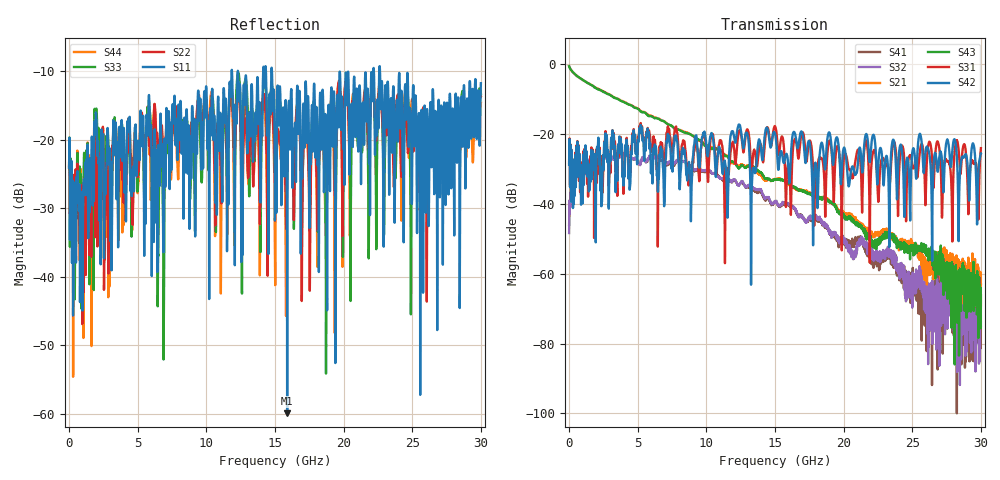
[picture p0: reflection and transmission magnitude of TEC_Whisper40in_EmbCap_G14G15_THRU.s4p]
! Tyco Electronics
! G14G15_THRU
!! PART DESCRIPTION: Whisper 40in Megtron 6 VLP-HVLP-VLP Channel, Embedded Capactior Connecter at one end, bulkhead 2.4mm test pts
!! MODEL DESCRIPTION: System 4-port S-parameter
!! MODEL STATUS: Measured
!! MODEL GEOMETRY: Channel Model
!! MODEL FREQUENCY RANGE: DC to 30.000 GHz in 10.000 MHz frequency steps
!! MODEL EDGE RATE LIMITATION: 12.500 ps (Using conservative 0.5/Fmax rule of thumb)
!! TIME-DOMAIN TRANSFORM CAUTIONS:
!! 1.) Do not simulate transient edge rates faster than the number listed above.  Edge rates faster than this number
!!  contain significant spectral content at frequencies above the model's highest frequency.
!! 2.) Even when simulating edge rates that are slower than the number listed above, be aware that the best time
!!  resolution possible with a direct iFFT is (1 / 2Fmax).  As a result, time resolution is typically not adequate
!!  for most time-domain simulations unless tricks such as windowing are used to minimize leakage and aliasing.
!! 3.) Because the model has a uniform frequency step, a direct iFFT will result in an impulse that that has a time
!!  length given by either (1 / Fstep) or (1 / 2Fstep), depending on the transform being used.  Care has been taken
!!  in selecting the frequency step to ensure a settled impulse response for the model.  Therefore, convolution with
!!  the model's impulse response should present no issues.  However, if directly concatenating s-parameter models
!!  in the frequency domain a user must either interpolate necessary interim frequencies or complete impulse response
!!  zero-padding.  Impulse response zero-padding is more difficult, but more accurate.
!! PORT DEFINITIONS:
!! Port  1  ----->  Side A  G14  Side B  <-----  Port  2
!! Port  3  ----->  Side A  G15  Side B  <-----  Port  4
! Point-to-Point link (differential)  !
! Connectors:  !
!  1: STRADA Whisper  !
! Materials:  !
!  Backplane: Megtron-6 HVLP  !
!  Daughtercard: Megtron-6 VLP  !
! Stack-up:  !
!  Backplane: 20 layers, 200mil thick  !
!  Daughtercard: 14 layers, 110mil thick  !
! Trace Length:  !
!  Backplane: 30in  !
!  Daightercards: 5in  !
! Trace Width:  !
!  Backplane: 7-9-7 mils  !
!  Daughtercards: 6-9-6 mils  !
! Geometry:  !
!  Backplane: Stripline  !
!  Daughtercards: Stripline  !
! Layer Connections:  !
!  Backplane: Layer 16, counterbored(~6mil stub)  !
!  Daughtercard: Layer 9, counterbored(~6mil stub)  !
! Freq. Range: 0 GHz - 30 GHz  !
! Note1: non-mixed-mode s-parameters  !
! Note2: channel includes 2.4mm test points  !
! Touchstone data
! Created: 02-Jul-2013 by IdEM R2011 (7.0.3)
# Hz S MA R 50
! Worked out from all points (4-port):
!   3000 points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, 10 MHz to 30 GHz, reference 50 ohm
!   strongest paths, dB at 10 MHz, 7.51 GHz, 15.01 GHz, 22.51 GHz, 30 GHz:
!     S42: -28.8, -29.7, -19.9, -30.1, -25.5
!     S31: -28.3, -24.8, -17.7, -38.8, -24.0
!     S43: -0.5, -17.7, -33.0, -51.0, -66.2
!     S21: -0.5, -17.7, -32.8, -48.0, -69.0
!     S32: -48.3, -28.3, -39.2, -56.2, -74.9
!     S41: -46.0, -28.6, -39.4, -55.4, -63.1
!   lowest |S11| = -59.9 dB at 15.89 GHz (marker M1), VSWR 1.00, Z = 50 - j0.101 ohm
!   |S11| at or under -10 dB: start of sweep to 11.85 GHz; 14.78 GHz to 22.17 GHz (7.385 GHz wide, 40 % of centre); 22.65 GHz to end of sweep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
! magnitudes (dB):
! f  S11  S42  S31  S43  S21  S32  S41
! 10 MHz  -24.1  -28.8  -28.3  -0.5  -0.5  -48.3  -46.0
! 3.91 GHz  -22.4  -32.3  -31.7  -10.6  -10.5  -25.6  -25.4
! 11.49 GHz  -23.1  -34.9  -30.1  -26.2  -26.1  -32.4  -32.7
! 12.31 GHz  -10.1  -17.9  -20.8  -29.4  -29.1  -34.5  -34.4
! 13.33 GHz  -12.6  -33.6  -31.1  -29.3  -29.6  -35.4  -35.7
! 15.89 GHz  -59.9  -26.1  -30.3  -33.7  -33.8  -40.0  -40.2
! 30 GHz  -11.8  -25.5  -24.0  -66.2  -69.0  -74.9  -63.1
